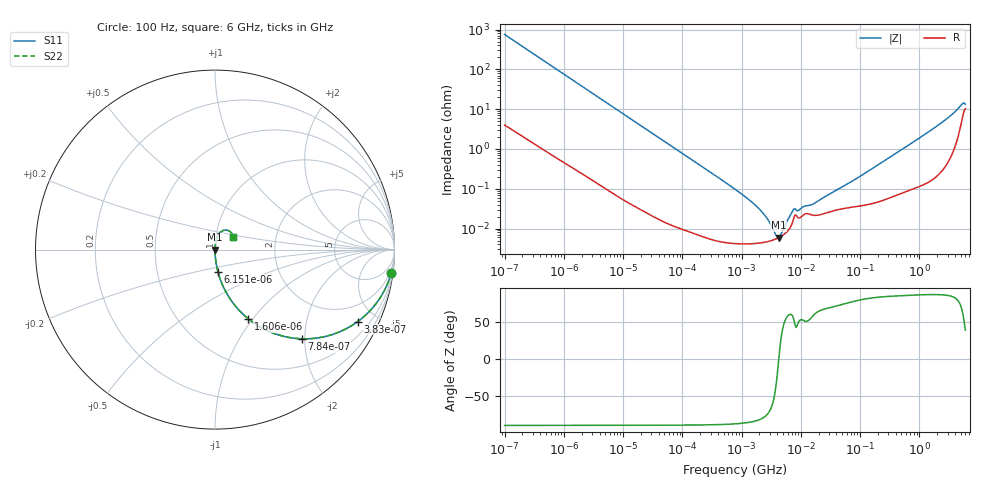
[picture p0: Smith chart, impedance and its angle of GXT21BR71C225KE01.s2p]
!Murata Part Number: GXT21BR71C225KE01
!These Parameters are Measured in Series Mode Connection
!Data Generated on Jan 08, 2026
!  o--ll--o
!Port1  Port2
!  o------o
!Operation Temp=25[degC], DC Bias Voltage=0[V]
!Freq. Start=100[Hz] Stop=6[GHz] 401[Steps]
# Hz S RI R 50
!Freq.(Hz) S11(Real) S11(Imag) S21(Real) S21(Imag) S12(Real) S12(Imag) S22(Real) S22(Imag)
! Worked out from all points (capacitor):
!   401 points, 100 Hz to 6 GHz, reference 50 ohm
!   read as one part in series: C = 2.11 uF near 109 Hz
!   lowest |Z| = 5.94 mohm at 4.246 MHz (marker M1)
!   series resonance near 4.242 MHz, so ESL is about 670 pH
!   S11 on the Smith chart (normalised r, x): 100 Hz: 1, -15; 383 Hz: 1.02, -3.96; 784 Hz: 1.01, -1.94; 1.606 kHz: 1.01, -0.95; 6.151 kHz: 1.00, -0.25; 6 GHz: 1.21, +0.17
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100  0.9821 -0.1301  0.0179 0.1301  0.0179 0.1301  0.9821 -0.1301
214  0.9246 -0.2613  0.0754 0.2613  0.0754 0.2613  0.9246 -0.2613
383  0.7951 -0.4008  0.2049 0.4008  0.2049 0.4008  0.7951 -0.4008
784  0.4843 -0.4968  0.5157 0.4968  0.5157 0.4968  0.4843 -0.4968
1606  0.1854 -0.3855  0.8146 0.3855  0.8146 0.3855  0.1854 -0.3855
2008  0.1276 -0.3305  0.8724 0.3305  0.8724 0.3305  0.1276 -0.3305
6151  0.0161 -0.1225  0.9839 0.1225  0.9839 0.1225  0.0161 -0.1225
40335  0.000534 -0.0191  0.9995 0.0191  0.9995 0.0191  0.000534 -0.0191
774597  4.29e-05 -0.000977  1 0.000977  1 0.000977  4.29e-05 -0.000977
1896632  4.3e-05 -0.000331  1 0.000331  1 0.000331  4.3e-05 -0.000331
2481164  4.55e-05 -0.000209  1 0.000209  1 0.000209  4.55e-05 -0.000209
3394479  5.15e-05 -8.39e-05  0.9999 8.39e-05  0.9999 8.39e-05  5.15e-05 -8.39e-05
4246196  5.94e-05 4e-07  0.9999 -4e-07  0.9999 -4e-07  5.94e-05 4e-07
4856642  6.67e-05 5.17e-05  0.9999 -5.17e-05  0.9999 -5.17e-05  6.67e-05 5.17e-05
5311619  7.35e-05 8.73e-05  0.9999 -8.73e-05  0.9999 -8.73e-05  7.35e-05 8.73e-05
7599586  0.000181 0.000246  0.9998 -0.000246  0.9998 -0.000246  0.000181 0.000246
1.555665e7  0.000219 0.000339  0.9998 -0.000339  0.9998 -0.000339  0.000219 0.000339
7.797396e7  0.000352 0.0016  0.9996 -0.0016  0.9996 -0.0016  0.000352 0.0016
3.124326e8  0.000622 0.00607  0.9994 -0.00607  0.9994 -0.00607  0.000622 0.00607
3.352442e9  0.0105 0.0667  0.9895 -0.0667  0.9895 -0.0667  0.0105 0.0667
5.016141e9  0.0497 0.1077  0.9503 -0.1077  0.9503 -0.1077  0.0497 0.1077
6e9  0.0987 0.0685  0.9013 -0.0685  0.9013 -0.0685  0.0987 0.0685
